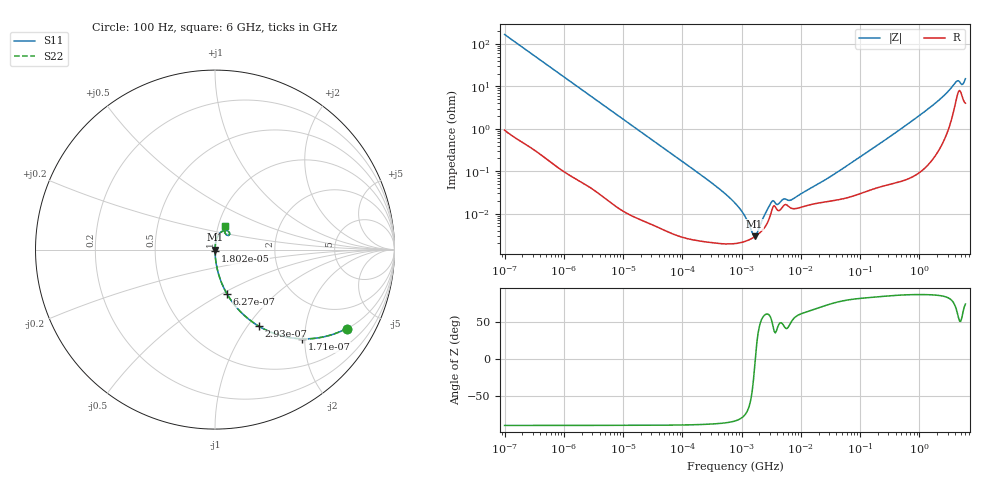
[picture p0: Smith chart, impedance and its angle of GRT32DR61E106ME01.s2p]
!Murata Part Number: GRT32DR61E106ME01
!These Parameters are Measured in Series Mode Connection
!Data Generated on Jun 19, 2026
!  o--ll--o
!Port1  Port2
!  o------o
!Operation Temp=25[degC], DC Bias Voltage=0[V]
!Freq. Start=100[Hz] Stop=6[GHz] 401[Steps]
# Hz S RI R 50
!Freq.(Hz) S11(Real) S11(Imag) S21(Real) S21(Imag) S12(Real) S12(Imag) S22(Real) S22(Imag)
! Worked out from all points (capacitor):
!   401 points, 100 Hz to 6 GHz, reference 50 ohm
!   read as one part in series: C = 9.57 uF near 109 Hz
!   lowest |Z| = 2.91 mohm at 1.658 MHz (marker M1)
!   series resonance near 1.703 MHz, so ESL is about 910 pH
!   S11 on the Smith chart (normalised r, x): 100 Hz: 1.02, -3.32; 171 Hz: 1.01, -1.94; 293 Hz: 1.01, -1.14; 627 Hz: 1.00, -0.53; 18.02 kHz: 1.00, -0.02; 6 GHz: 1.08, +0.29
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100  0.733 -0.4396  0.267 0.4396  0.267 0.4396  0.733 -0.4396
171  0.4861 -0.497  0.5139 0.497  0.5139 0.497  0.4861 -0.497
293  0.2461 -0.4278  0.7539 0.4278  0.7539 0.4278  0.2461 -0.4278
627  0.0677 -0.2483  0.9323 0.2483  0.9323 0.2483  0.0677 -0.2483
2008  0.00748 -0.0829  0.9925 0.0829  0.9925 0.0829  0.00748 -0.0829
18016  0.000164 -0.0094  0.9998 0.0094  0.9998 0.0094  0.000164 -0.0094
40335  6.43e-05 -0.00421  0.9999 0.00421  0.9999 0.00421  6.43e-05 -0.00421
330837  2.08e-05 -0.0005  1 0.0005  1 0.0005  2.08e-05 -0.0005
774597  1.98e-05 -0.000177  1 0.000177  1 0.000177  1.98e-05 -0.000177
1108252  2.19e-05 -9.06e-05  1 9.06e-05  1 9.06e-05  2.19e-05 -9.06e-05
1658239  2.86e-05 -5.5e-06  1 5.5e-06  1 5.5e-06  2.86e-05 -5.5e-06
2372521  4.48e-05 7.34e-05  1 -7.34e-05  1 -7.34e-05  4.48e-05 7.34e-05
3245845  0.000121 0.000151  0.9999 -0.000151  0.9999 -0.000151  0.000121 0.000151
4060267  0.00012 0.000113  0.9999 -0.000113  0.9999 -0.000113  0.00012 0.000113
5079039  0.000153 0.000159  0.9998 -0.000159  0.9998 -0.000159  0.000153 0.000159
6948629  0.000134 0.000165  0.9999 -0.000165  0.9999 -0.000165  0.000134 0.000165
1.555665e7  0.000167 0.000382  0.9998 -0.000382  0.9998 -0.000382  0.000167 0.000382
3.124326e8  0.000527 0.00638  0.9995 -0.00638  0.9995 -0.00638  0.000527 0.00638
1.791126e9  0.00358 0.038  0.9964 -0.038  0.9964 -0.038  0.00358 0.038
4.193612e9  0.0577 0.1069  0.9423 -0.1069  0.9423 -0.1069  0.0577 0.1069
5.245841e9  0.064 0.0808  0.936 -0.0808  0.936 -0.0808  0.064 0.0808
6e9  0.057 0.1318  0.943 -0.1318  0.943 -0.1318  0.057 0.1318
